(* Logix 5000 AddOnInstructionDefinition export Banner_IOL_Generic_Param_v4; software revision 33.00 *)

TYPE Banner_IOL_Generic_v4 :
STRUCT
   Index : INT;   // Value of Index to read/write.
   Sub_Index : INT;   // Value of Sub-Index to read/write.
   Data_Length : INT;   // Length (in bytes) for the data.
   Activate : BOOL;   // True starts the read or write of parameter from an IO-Link device.
   RW : BOOL;   // False = Read, True = Write.
   Busy : BOOL;
   Done : BOOL;
   Reset : BOOL;
   Clear_Data : BOOL;
   Data : SINT[180];
END_STRUCT
END_TYPE

TYPE Banner_IOL_Port_v4 :   // UDT that has all of the data items necessary to communicate with a specific Port on a IO-Link Master
STRUCT
   Port_Controlled : INT;   // Each bit represents a port on an IO-Link Master. Set to 1 to tell AOI to control that port.
   Port_Activate : INT;   // Each bit represents a port on an IO-Link Master. When ON that port will process any commands in queue.
   Port_Read : INT;   // Each bit represents a port on an IO-Link Master. Used to determine when device AOI has requested a Read command.
   Port_Write : INT;   // Each bit represents a port on an IO-Link Master. Used to determine when device AOI has requested a Write command.
   Port_RW_Complete : INT;   // Each bit represents a port on an IO-Link Master. Tells device AOI that Read or Write request has been completed.
   Port_Device_Read : INT;
   Data_Transfer : SINT[190];   // Array to transfer data from IO-Master to device AOIs.
END_STRUCT
END_TYPE

ADD_ON_INSTRUCTION Banner_IOL_Generic_Param_v4   (* revision 4.0, vendor Banner Engineering *)
// AOI to read and write parameter generic IO-Link parameter data.
// Sub-Index access not possible at this time.
VAR_IN_OUT
   IOL : Banner_IOL_Generic_v4; {required}
   Port_Data : Banner_IOL_Port_v4; {required}
END_VAR
VAR_INPUT
   Port : DINT; {required}
END_VAR
VAR
   Local_Control : DINT; {access None}
   Command_Being_Processed : BOOL; {access None}
END_VAR

ROUTINE Logic   (* ladder *)
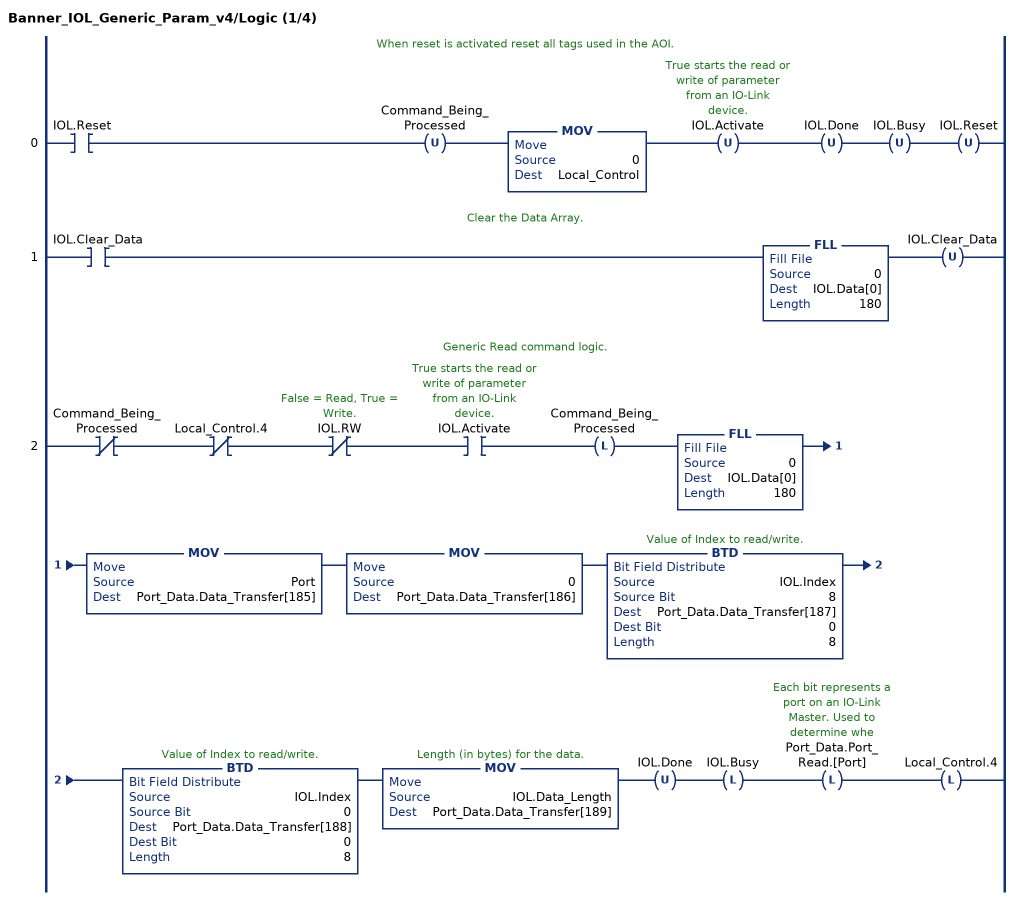
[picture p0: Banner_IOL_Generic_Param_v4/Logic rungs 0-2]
   // When reset is activated reset all tags used in the AOI.
   0: XIC(IOL.Reset)OTU(Command_Being_Processed)MOV(0,Local_Control)OTU(IOL.Activate)OTU(IOL.Done)OTU(IOL.Busy)OTU(IOL.Reset);
   // Clear the Data Array.
   1: XIC(IOL.Clear_Data)FLL(0,IOL.Data[0],180)OTU(IOL.Clear_Data);
   // Generic Read command logic.
   2: XIO(Command_Being_Processed)XIO(Local_Control.4)XIO(IOL.RW)XIC(IOL.Activate)OTL(Command_Being_Processed)FLL(0,IOL.Data[0],180)MOV(Port,Port_Data.Data_Transfer[185])MOV(0,Port_Data.Data_Transfer[186])BTD(IOL.Index,8,Port_Data.Data_Transfer[187],0,8)BTD(IOL.Index,0,Port_Data.Data_Transfer[188],0,8)MOV(IOL.Data_Length,Port_Data.Data_Transfer[189])OTU(IOL.Done)OTL(IOL.Busy)OTL(Port_Data.Port_Read.[Port])OTL(Local_Control.4);
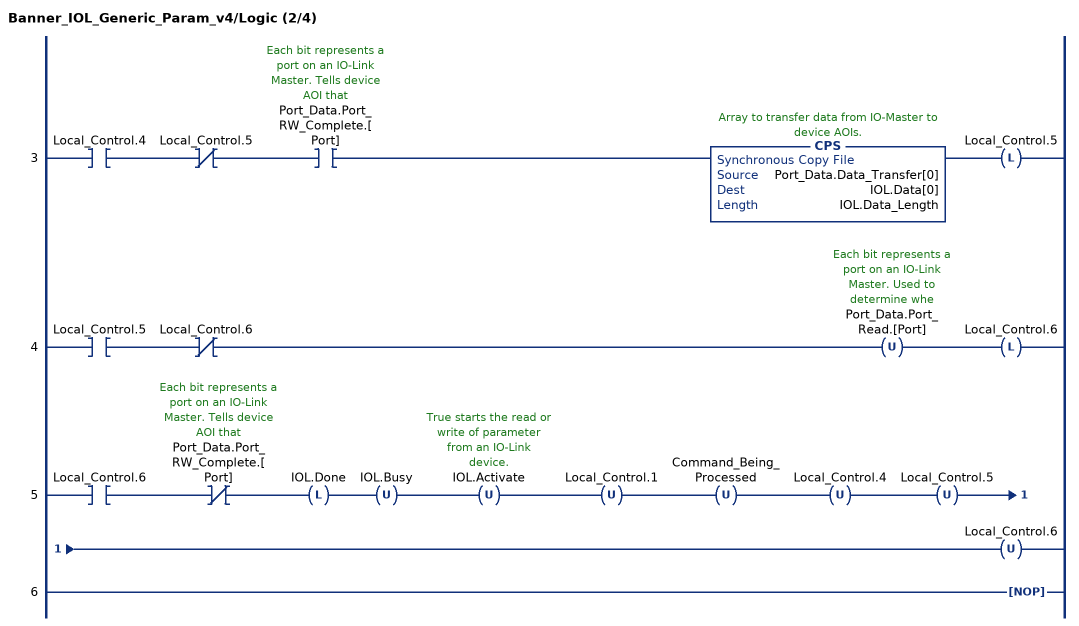
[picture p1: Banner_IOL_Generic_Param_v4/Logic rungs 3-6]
   3: XIC(Local_Control.4)XIO(Local_Control.5)XIC(Port_Data.Port_RW_Complete.[Port])CPS(Port_Data.Data_Transfer[0],IOL.Data[0],IOL.Data_Length)OTL(Local_Control.5);
   4: XIC(Local_Control.5)XIO(Local_Control.6)OTU(Port_Data.Port_Read.[Port])OTL(Local_Control.6);
   5: XIC(Local_Control.6)XIO(Port_Data.Port_RW_Complete.[Port])OTL(IOL.Done)OTU(IOL.Busy)OTU(IOL.Activate)OTU(Local_Control.1)OTU(Command_Being_Processed)OTU(Local_Control.4)OTU(Local_Control.5)OTU(Local_Control.6);
   6: NOP();
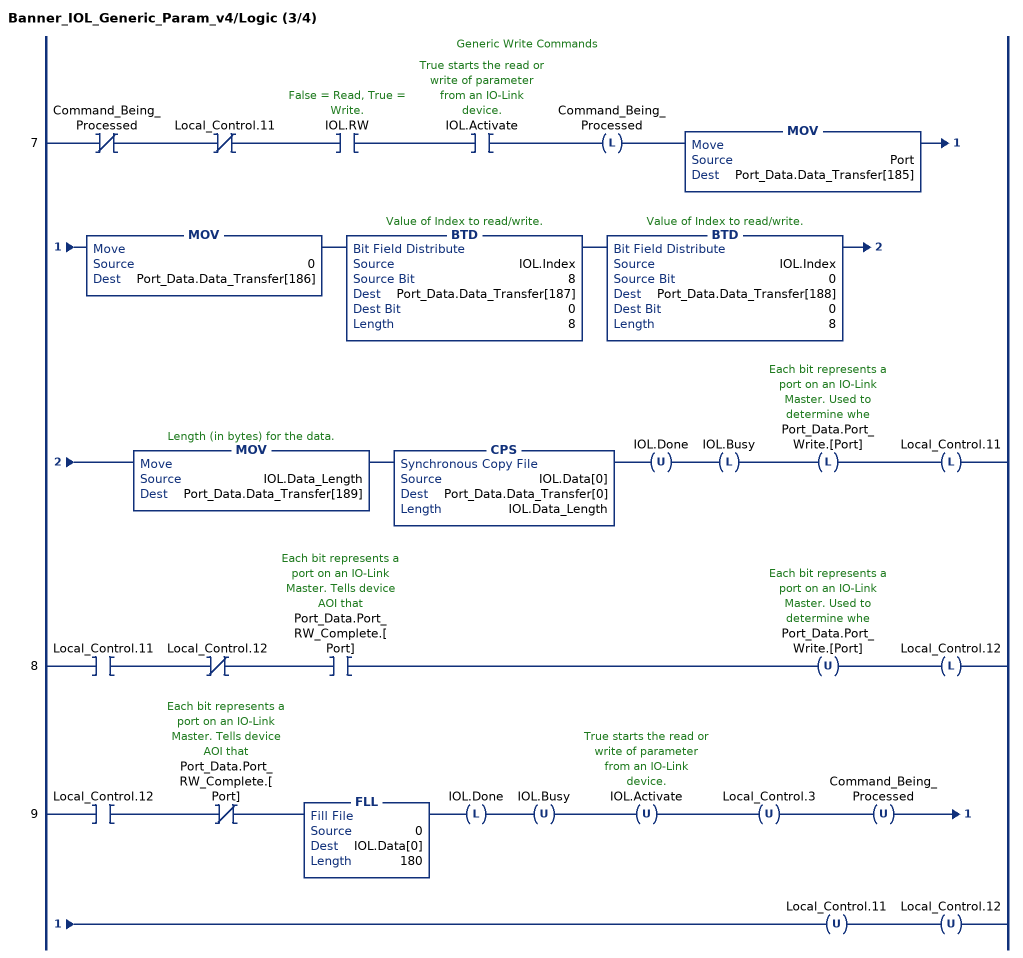
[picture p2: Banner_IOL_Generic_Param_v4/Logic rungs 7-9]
   // Generic Write Commands
   7: XIO(Command_Being_Processed)XIO(Local_Control.11)XIC(IOL.RW)XIC(IOL.Activate)OTL(Command_Being_Processed)MOV(Port,Port_Data.Data_Transfer[185])MOV(0,Port_Data.Data_Transfer[186])BTD(IOL.Index,8,Port_Data.Data_Transfer[187],0,8)BTD(IOL.Index,0,Port_Data.Data_Transfer[188],0,8)MOV(IOL.Data_Length,Port_Data.Data_Transfer[189])CPS(IOL.Data[0],Port_Data.Data_Transfer[0],IOL.Data_Length)OTU(IOL.Done)OTL(IOL.Busy)OTL(Port_Data.Port_Write.[Port])OTL(Local_Control.11);
   8: XIC(Local_Control.11)XIO(Local_Control.12)XIC(Port_Data.Port_RW_Complete.[Port])OTU(Port_Data.Port_Write.[Port])OTL(Local_Control.12);
   9: XIC(Local_Control.12)XIO(Port_Data.Port_RW_Complete.[Port])FLL(0,IOL.Data[0],180)OTL(IOL.Done)OTU(IOL.Busy)OTU(IOL.Activate)OTU(Local_Control.3)OTU(Command_Being_Processed)OTU(Local_Control.11)OTU(Local_Control.12);
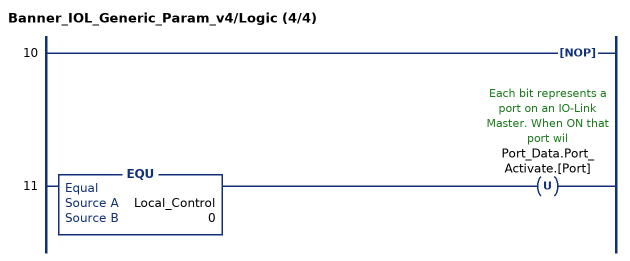
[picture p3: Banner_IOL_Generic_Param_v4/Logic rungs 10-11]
   10: NOP();
   11: EQU(Local_Control,0)OTU(Port_Data.Port_Activate.[Port]);
END_ROUTINE
END_ADD_ON_INSTRUCTION
